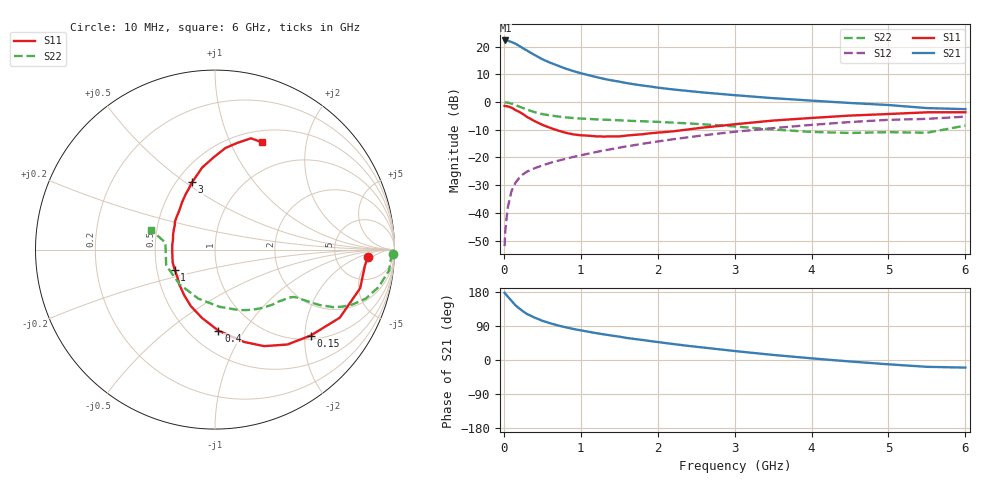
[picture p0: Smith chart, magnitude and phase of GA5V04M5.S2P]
! Infineon Technologies  Discrete & RF Semiconductors
! BF775
! Si NPN RF Bipolar Junction Transistor in SOT23
! VCE = 5 V  IC = 4.5 mA
! Common Emitter S-Parameters:  May  1996
# GHz  S  MA  R  50
!  f  S11  S21  S12  S22
! GHz  MAG  ANG  MAG  ANG  MAG  ANG  MAG  ANG
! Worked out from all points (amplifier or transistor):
!   36 points, 10 MHz to 6 GHz, reference 50 ohm
!   highest |S21| = 22.2 dB at 20 MHz (marker M1)
!   |S21| within 3 dB of that: start of sweep to 260.8 MHz
!   unconditionally stable (mu >= 1): 851.9 MHz to 3.22 GHz
!   at 250 MHz: K = 0.45, MSG = 22.7 dB, |S12| = -26.1 dB
!   at 1.4 GHz: K = 1.12, MAG = 10.4 dB, |S12| = -17.0 dB
!   at 6 GHz: K = 0.94, MSG = 1.4 dB, |S12| = -5.3 dB
!   S11 on the Smith chart (normalised r, x): 10 MHz: 11, -4; 150 MHz: 1.09, -2.14; 400 MHz: 0.68, -0.77; 1 GHz: 0.62, -0.15; 3 GHz: 0.60, +0.53; 6 GHz: 0.63, +1.32
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0.01  0.8524 -2.9  12.86 177.5  0.0025 95.2  0.9936 -1.3
0.02  0.8407 -5.8  12.92 174.7  0.0049 87.4  0.9819 -2.7
0.05  0.8367 -14.9  12.83 167.5  0.0123 82.8  0.9768 -6.8
0.1  0.7922 -28.6  12.1 156.2  0.0248 75.0  0.9358 -12.8
0.15  0.7167 -41.9  11.31 144.6  0.0346 69.3  0.8835 -18.0
0.2  0.6649 -52.7  10.31 136.1  0.0427 64.5  0.8271 -21.6
0.25  0.6035 -63.0  9.332 128.4  0.0497 61.4  0.7765 -24.2
0.3  0.5401 -72.4  8.494 121.6  0.0555 59.2  0.731 -26.0
0.4  0.4517 -87.6  7.07 111.9  0.0637 56.6  0.6566 -28.0
0.5  0.3879 -100.7  5.923 103.6  0.0717 55.7  0.6059 -28.9
0.6  0.3427 -113.1  5.143 97.1  0.0796 55.6  0.5738 -29.5
0.7  0.307 -123.9  4.542 91.4  0.0868 55.6  0.5489 -30.0
0.8  0.2797 -134.9  4.023 86.5  0.094 56.1  0.5288 -30.4
1  0.251 -153.4  3.311 78.2  0.1093 57.0  0.5037 -31.7
1.1  0.2466 -163.1  3.053 74.6  0.117 57.2  0.4947 -32.7
1.6  0.2482 160.1  2.191 58.2  0.1587 57.0  0.4607 -38.6
2.2  0.2954 132.3  1.685 42.2  0.2127 54.3  0.4248 -48.9
3  0.3967 108.7  1.33 23.7  0.2899 47.6  0.3626 -68.4
3.5  0.4626 98.9  1.174 13.4  0.3377 42.1  0.3194 -85.6
4.5  0.5691 84.1  0.961 -3.9  0.4349 29.7  0.2761 -135.5
5.5  0.6516 72.1  0.777 -18.0  0.4963 14.5  0.2789 172.0
6  0.6527 66.6  0.744 -20.1  0.5444 10.2  0.3753 162.7
